DATA_BLOCK DB 4
TITLE =BLOCK DATA FOR TIMER PLC - OP37
AUTHOR : Esposito
FAMILY : EGAL_srl
NAME : DB_SERVI
VERSION : 0.1


  STRUCT
   Over_fault_1 : WORD ;	//Error of conversion FC_105 for PEW288 Overload trasducer
   Over_fault_2 : WORD ;	//Error of conversion FC_105 for PEW290 Overload trasducer
   Over_fault_3 : WORD ;	//Error of conversion FC_105 for PEW292 Overload trasducer
   Over_fault_4 : WORD ;	//Error of conversion FC_105 for PEW294 Overload trasducer
   Over_fault_5 : WORD ;	//Error of conversion FC_105 for PEW296 Overload proportional valve
   Over_fault_6 : WORD ;	//Error of conversion FC_106 for PAW304 Overload proportional valve
   Bala_fault_1 : WORD ;	//Error of conversion FC_105 for PEW298 Balancing trasducer
   Spare_1 : WORD ;	//Spare for program
   Spare_2 : WORD ;	//Spare for program
   Moto_fault_1 : WORD ;	//Error of conversion FC_105 for PEW300 Main motor press
   Moto_fault_2 : WORD ;	//Error of conversion FC_105 for PEW302 Main motor press
   Moto_fault_3 : WORD ;	//Error of conversion FC_106 for PAW306 Main motor press
   Serv_byte_A : WORD ;	//Support for byte of alarm PLC automation
   Bala_fault_2 : WORD ;	//Error of conversion FC_105 for scale value Balancing
   Bala_fault_3 : WORD ;	//Error of conversion FC_105 for scale value Balancing
   Balanc_value_R : REAL ;
   SEN_RES_SFB : BOOL ;
   SEN_RES_SFB1 : BOOL ;
   SEN_RES_SFB2 : BOOL ;
   SEN_RES_SFB3 : BOOL ;
   SEN_RES_SFB4 : BOOL ;
   SEN_RES_SFB5 : BOOL ;
   SEN_RES_SFB6 : BOOL ;
   SEN_RES_SFB7 : BOOL ;
   SEN_RES_SFB8 : BOOL ;
   SEN_RES_SFB9 : BOOL ;
   SEN_RES_SFB10 : BOOL ;
   SEN_RES_SFB11 : BOOL ;
   SEN_RES_SFB12 : BOOL ;
   SEN_RES_SFB13 : BOOL ;
   SEN_RES_SFB14 : BOOL ;
   SEN_RES_SFB15 : BOOL ;
   SEN_REC_RETVAL : INT ;
   SEN_REC_VALUE : DWORD ;
   SEN_REC_DATA : DWORD ;
   VALUE_OPSCHUIF : DINT ;
   VALUE_ROB1 : WORD ;
   VALUE_ROB1_1 : DWORD ;
  END_STRUCT ;
BEGIN
   Over_fault_1 := W#16#0;
   Over_fault_2 := W#16#0;
   Over_fault_3 := W#16#0;
   Over_fault_4 := W#16#0;
   Over_fault_5 := W#16#0;
   Over_fault_6 := W#16#0;
   Bala_fault_1 := W#16#0;
   Spare_1 := W#16#0;
   Spare_2 := W#16#0;
   Moto_fault_1 := W#16#0;
   Moto_fault_2 := W#16#0;
   Moto_fault_3 := W#16#0;
   Serv_byte_A := W#16#0;
   Bala_fault_2 := W#16#0;
   Bala_fault_3 := W#16#0;
   Balanc_value_R := 0.000000e+000;
   SEN_RES_SFB := FALSE;
   SEN_RES_SFB1 := FALSE;
   SEN_RES_SFB2 := FALSE;
   SEN_RES_SFB3 := FALSE;
   SEN_RES_SFB4 := FALSE;
   SEN_RES_SFB5 := FALSE;
   SEN_RES_SFB6 := FALSE;
   SEN_RES_SFB7 := FALSE;
   SEN_RES_SFB8 := FALSE;
   SEN_RES_SFB9 := FALSE;
   SEN_RES_SFB10 := FALSE;
   SEN_RES_SFB11 := FALSE;
   SEN_RES_SFB12 := FALSE;
   SEN_RES_SFB13 := FALSE;
   SEN_RES_SFB14 := FALSE;
   SEN_RES_SFB15 := FALSE;
   SEN_REC_RETVAL := 0;
   SEN_REC_VALUE := DW#16#0;
   SEN_REC_DATA := DW#16#0;
   VALUE_OPSCHUIF := L#0;
   VALUE_ROB1 := W#16#0;
   VALUE_ROB1_1 := DW#16#0;
END_DATA_BLOCK

